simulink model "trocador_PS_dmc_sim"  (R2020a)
settings: Solver=VariableStepAuto  StartTime=0.0  StopTime=tsim  MaxStep=0.01  RelTol=1e-3
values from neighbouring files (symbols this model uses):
  F = f(1+N1:1+N2,:)    [diofantina.m]    (also in diofantinaC.m = f(1+N1:1+N2,1:nF); simEstudoInstavel_2.m = tf(0,1,Ts); simEstudoInstavel_1.m = tf(0,1,Ts); sim_3.m = tf(0,1,Ts))
  H = 2*(G'*Qy*G+Qu)    [tempo_insuficiente.m]    (also in ex_gpc_acaoatrasada2.m = zeros(Ny,nb+d); ex_gpc_acaoatrasada.m = zeros(Ny,nb+d); tempo_insuficiente2.m; simEstudoInstavel_2.m = H1-H2)
  tpert = 15    [trocador_PS_dmc_dtc.m]
  tref = 4    [trocador_PS_dmc_dtc.m]
  Ts = 0.15    [trocador_PS_dmc_dtc.m]    (also in dtc_dmc_agua_metanol.m = 1; tempo_insuficiente.m = 1; ex_warmstart.m = 0.1; ex_rest_inversa_comp.m = 0.1)
undefined symbols (not defined in the file or in its folder): amppert, ampref, Kgpc1, zr
libraries: cstblocks x3

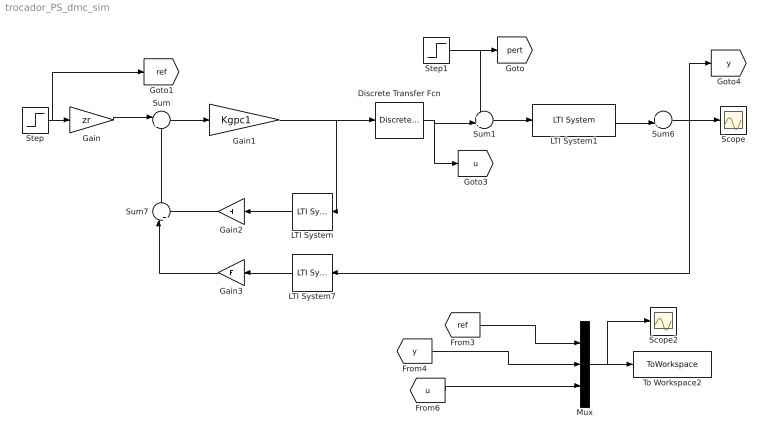
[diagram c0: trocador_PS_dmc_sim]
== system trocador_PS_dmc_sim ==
  Discrete Transfer Fcn : DiscreteTransferFcn  Numerator=[1 0]  Denominator=[1 -1]  SampleTime=Ts
  Gain : Gain  Gain=zr  Multiplication=Matrix(K*u)
  Gain1 : Gain  Gain=Kgpc1  Multiplication=Matrix(K*u)
  Gain2 : Gain  Gain=H  Multiplication=Matrix(K*u)
  Gain3 : Gain  Gain=F  Multiplication=Matrix(K*u)
  LTI System : cstblocks/LTI System  sys=zu  IC=[]
  LTI System1 : cstblocks/LTI System  sys=P  IC=[]
  LTI System7 : cstblocks/LTI System  sys=zy  IC=[]
  Mux : Mux  Inputs=3
  Scope : Scope
  Scope2 : Scope
  Step : Step  Time=tref  After=ampref  SampleTime=0
  Step1 : Step  Time=tpert  After=amppert  SampleTime=0
  Sum : Sum  Inputs=|+-
  Sum1 : Sum  Inputs=++|
  Sum6 : Sum  Inputs=++|
  Sum7 : Sum  Inputs=|++
  To Workspace2 : ToWorkspace  VariableName=simout  SampleTime=-1
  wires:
  Step/1 -> [ref], Gain/1
  Sum/1 -> Gain1/1
  Gain1/1 -> LTI System/1, Discrete Transfer Fcn/1
  Step1/1 -> Sum1/1, [pert]
  Sum1/1 -> LTI System1/1
  Mux/1 -> Scope2/1, To Workspace2/1
  [ref] -> Mux/1
  [y] -> Mux/2
  LTI System1/1 -> Sum6/2
  Sum6/1 -> LTI System7/1, [y], Scope/1
  Gain/1 -> Sum/1
  Discrete Transfer Fcn/1 -> [u], Sum1/2
  Sum7/1 -> Sum/2
  Gain2/1 -> Sum7/2
  LTI System/1 -> Gain2/1
  Gain3/1 -> Sum7/1
  LTI System7/1 -> Gain3/1
  [u] -> Mux/3
